| / 7\'7   Xilinx XC4000XV I/O Buffer IBIS File
| \ \   Xilinx Inc.
| / /   2100 Logic Drive
| \_\/.\   San Jose,   CA 95124
| IBIS file xc4kxv.ibs created by s2ibis2 version 1.1
| North Carolina State University Electronics Research Laboratory  1995
[IBIS ver]   2.1
[File name]   xc4kxv.ibs
[File Rev]   1.1
[Date]   Dec. 11, 1998
[Source]   Spice netlist
[Notes]   - Best/worse process data included in this ibis model
   - Control flag setting:
   SLW=0 - fast slew rate
   SLW=1 - slow slew rate
   PCI=0 - driving 3.3V PCI bus
   PCI=1 - driving 5.0V PCI bus
   5VT=0 - 5.0V tolerant input off
   5VT=1 - 5.0V tolerant input on
   - Created by Joey Jia x4437
[Disclaimer] The data in this model is derived from SPICE simulations
   using modeling information extracted from the target pro-
   cess. While a great deal of care has been take to provide
   information that is accurate, this model is considered
   preliminary as it has not been verified by actual silicon
   measurement. Treat the data in this model as preliminary
   until actual silicon verification is performed.
[Copyright]   Xilinx Inc. All right reserved
|   Component XC40110XV_BG325[SLW=0;PCI=0;5VT=0]
[Component]   XC40110XV_BG325[SLW=0;PCI=0;5VT=0]
[Manufacturer]   Xilinx Inc.
[Package]
| variable   typ   min   max
R_pkg   0.206   0.146   0.267
L_pkg   4.950nH   3.300nH   6.600nH
C_pkg   0.885pF   0.650pF   1.120pF
[Pin]  signal_name   model_name   R_pin   L_pin   C_pin
io   iob   IO_000   NA   NA   NA
|   Component XC40110XV_BG325[SLW=0;PCI=0;5VT=1]
[Component]   XC40110XV_BG325[SLW=0;PCI=0;5VT=1]
[Manufacturer]   Xilinx Inc.
[Package]
| variable   typ   min   max
R_pkg   0.206   0.146   0.267
L_pkg   4.950nH   3.300nH   6.600nH
C_pkg   0.885pF   0.650pF   1.120pF
[Pin]  signal_name   model_name   R_pin   L_pin   C_pin
io   iob   IO_001   NA   NA   NA
|   Component XC40110XV_BG325[SLW=0;PCI=1;5VT=0]
[Component]   XC40110XV_BG325[SLW=0;PCI=1;5VT=0]
[Manufacturer]   Xilinx Inc.
[Package]
| variable   typ   min   max
R_pkg   0.206   0.146   0.267
L_pkg   4.950nH   3.300nH   6.600nH
C_pkg   0.885pF   0.650pF   1.120pF
[Pin]  signal_name   model_name   R_pin   L_pin   C_pin
io   iob   IO_010   NA   NA   NA
|   Component XC40110XV_BG325[SLW=0;PCI=1;5VT=1]
[Component]   XC40110XV_BG325[SLW=0;PCI=1;5VT=1]
[Manufacturer]   Xilinx Inc.
[Package]
| variable   typ   min   max
R_pkg   0.206   0.146   0.267
L_pkg   4.950nH   3.300nH   6.600nH
C_pkg   0.885pF   0.650pF   1.120pF
[Pin]  signal_name   model_name   R_pin   L_pin   C_pin
io   iob   IO_011   NA   NA   NA
|   Component XC40110XV_BG325[SLW=1;PCI=0;5VT=0]
[Component]   XC40110XV_BG325[SLW=1;PCI=0;5VT=0]
[Manufacturer]   Xilinx Inc.
[Package]
| variable   typ   min   max
R_pkg   0.206   0.146   0.267
L_pkg   4.950nH   3.300nH   6.600nH
C_pkg   0.885pF   0.650pF   1.120pF
[Pin]  signal_name   model_name   R_pin   L_pin   C_pin
io   iob   IO_100   NA   NA   NA
|   Component XC40110XV_BG325[SLW=1;PCI=0;5VT=1]
[Component]   XC40110XV_BG325[SLW=1;PCI=0;5VT=1]
[Manufacturer]   Xilinx Inc.
[Package]
| variable   typ   min   max
R_pkg   0.206   0.146   0.267
L_pkg   4.950nH   3.300nH   6.600nH
C_pkg   0.885pF   0.650pF   1.120pF
[Pin]  signal_name   model_name   R_pin   L_pin   C_pin
io   iob   IO_101   NA   NA   NA
|   Component XC40110XV_BG325[SLW=1;PCI=1;5VT=0]
[Component]   XC40110XV_BG325[SLW=1;PCI=1;5VT=0]
[Manufacturer]   Xilinx Inc.
[Package]
| variable   typ   min   max
R_pkg   0.206   0.146   0.267
L_pkg   4.950nH   3.300nH   6.600nH
C_pkg   0.885pF   0.650pF   1.120pF
[Pin]  signal_name   model_name   R_pin   L_pin   C_pin
io   iob   IO_110   NA   NA   NA
|   Component XC40110XV_BG325[SLW=1;PCI=1;5VT=1]
[Component]   XC40110XV_BG325[SLW=1;PCI=1;5VT=1]
[Manufacturer]   Xilinx Inc.
[Package]
| variable   typ   min   max
R_pkg   0.206   0.146   0.267
L_pkg   4.950nH   3.300nH   6.600nH
C_pkg   0.885pF   0.650pF   1.120pF
[Pin]  signal_name   model_name   R_pin   L_pin   C_pin
io   iob   IO_111   NA   NA   NA
|+++++++++++++++++++++++++++++++++++++++++++++++++++++++++++++++++++++++++
|   Component XC40110XV_BG432[SLW=0;PCI=0;5VT=0]
[Component]   XC40110XV_BG432[SLW=0;PCI=0;5VT=0]
[Manufacturer]   Xilinx Inc.
[Package]
| variable   typ   min   max
R_pkg   249.500m   187.000m   312.000m
L_pkg   6.200nH   4.500nH   7.900nH
C_pkg   1.100pF   0.850pF   1.350pF
[Pin]  signal_name   model_name   R_pin   L_pin   C_pin
io   iob   IO_000   NA   NA   NA
| End [Component] XC40110XV_BG432[SLW=0;PCI=0;5VT=0]
|   Component XC40110XV_BG432[SLW=0;PCI=0;5VT=1]
[Component]   XC40110XV_BG432[SLW=0;PCI=0;5VT=1]
[Manufacturer]   Xilinx Inc.
[Package]
| variable   typ   min   max
R_pkg   249.500m   187.000m   312.000m
L_pkg   6.200nH   4.500nH   7.900nH
C_pkg   1.100pF   0.850pF   1.350pF
[Pin]  signal_name   model_name   R_pin   L_pin   C_pin
io   iob   IO_001   NA   NA   NA
| End [Component] XC40110XV_BG432[SLW=0;PCI=0;5VT=1]
|   Component XC40110XV_BG432[SLW=0;PCI=1;5VT=0]
[Component]   XC40110XV_BG432[SLW=0;PCI=1;5VT=0]
[Manufacturer]   Xilinx Inc.
[Package]
| variable   typ   min   max
R_pkg   249.500m   187.000m   312.000m
L_pkg   6.200nH   4.500nH   7.900nH
C_pkg   1.100pF   0.850pF   1.350pF
[Pin]  signal_name   model_name   R_pin   L_pin   C_pin
io   iob   IO_010   NA   NA   NA
| End [Component] XC40110XV_BG432[SLW=0;PCI=1;5VT=0]
|   Component XC40110XV_BG432[SLW=0;PCI=1;5VT=1]
[Component]   XC40110XV_BG432[SLW=0;PCI=1;5VT=1]
[Manufacturer]   Xilinx Inc.
[Package]
| variable   typ   min   max
R_pkg   249.500m   187.000m   312.000m
L_pkg   6.200nH   4.500nH   7.900nH
C_pkg   1.100pF   0.850pF   1.350pF
[Pin]  signal_name   model_name   R_pin   L_pin   C_pin
io   iob   IO_011   NA   NA   NA
| End [Component] XC40110XV_BG432[SLW=0;PCI=1;5VT=1]
|   Component XC40110XV_BG432[SLW=1;PCI=0;5VT=0]
[Component]   XC40110XV_BG432[SLW=1;PCI=0;5VT=0]
[Manufacturer]   Xilinx Inc.
[Package]
| variable   typ   min   max
R_pkg   249.500m   187.000m   312.000m
L_pkg   6.200nH   4.500nH   7.900nH
C_pkg   1.100pF   0.850pF   1.350pF
[Pin]  signal_name   model_name   R_pin   L_pin   C_pin
io   iob   IO_100   NA   NA   NA
| End [Component] XC40110XV_BG432[SLW=1;PCI=0;5VT=0]
|   Component XC40110XV_BG432[SLW=1;PCI=0;5VT=1]
[Component]   XC40110XV_BG432[SLW=1;PCI=0;5VT=1]
[Manufacturer]   Xilinx Inc.
[Package]
| variable   typ   min   max
R_pkg   249.500m   187.000m   312.000m
L_pkg   6.200nH   4.500nH   7.900nH
C_pkg   1.100pF   0.850pF   1.350pF
[Pin]  signal_name   model_name   R_pin   L_pin   C_pin
io   iob   IO_101   NA   NA   NA
| End [Component] XC40110XV_BG432[SLW=1;PCI=0;5VT=1]
|   Component XC40110XV_BG432[SLW=1;PCI=1;5VT=0]
[Component]   XC40110XV_BG432[SLW=1;PCI=1;5VT=0]
[Manufacturer]   Xilinx Inc.
[Package]
| variable   typ   min   max
R_pkg   249.500m   187.000m   312.000m
L_pkg   6.200nH   4.500nH   7.900nH
C_pkg   1.100pF   0.850pF   1.350pF
[Pin]  signal_name   model_name   R_pin   L_pin   C_pin
io   iob   IO_110   NA   NA   NA
| End [Component] XC40110XV_BG432[SLW=1;PCI=1;5VT=0]
|   Component XC40110XV_BG432[SLW=1;PCI=1;5VT=1]
[Component]   XC40110XV_BG432[SLW=1;PCI=1;5VT=1]
[Manufacturer]   Xilinx Inc.
[Package]
| variable   typ   min   max
R_pkg   249.500m   187.000m   312.000m
L_pkg   6.200nH   4.500nH   7.900nH
C_pkg   1.100pF   0.850pF   1.350pF
[Pin]  signal_name   model_name   R_pin   L_pin   C_pin
io   iob   IO_111   NA   NA   NA
| End [Component] XC40110XV_BG432[SLW=1;PCI=1;5VT=1]
|+++++++++++++++++++++++++++++++++++++++++++++++++++++++++++++++++++++++++
|   Component XC40110XV_BG560[SLW=0;PCI=0;5VT=0]
[Component]   XC40110XV_BG560[SLW=0;PCI=0;5VT=0]
[Manufacturer]   Xilinx Inc.
[Package]
| variable   typ   min   max
R_pkg   247.500m   172.000m   323.000m
L_pkg   6.150nH   4.100nH   8.200nH
C_pkg   1.090pF   0.780pF   1.400pF
[Pin]  signal_name   model_name   R_pin   L_pin   C_pin
io   iob   IO_000   NA   NA   NA
| End [Component] XC40110XV_BG560[SLW=0;PCI=0;5VT=0]
|   Component XC40110XV_BG560[SLW=0;PCI=0;5VT=1]
[Component]   XC40110XV_BG560[SLW=0;PCI=0;5VT=1]
[Manufacturer]   Xilinx Inc.
[Package]
| variable   typ   min   max
R_pkg   247.500m   172.000m   323.000m
L_pkg   6.150nH   4.100nH   8.200nH
C_pkg   1.090pF   0.780pF   1.400pF
[Pin]  signal_name   model_name   R_pin   L_pin   C_pin
io   iob   IO_001   NA   NA   NA
| End [Component] XC40110XV_BG560[SLW=0;PCI=0;5VT=1]
|   Component XC40110XV_BG560[SLW=0;PCI=1;5VT=0]
[Component]   XC40110XV_BG560[SLW=0;PCI=1;5VT=0]
[Manufacturer]   Xilinx Inc.
[Package]
| variable   typ   min   max
R_pkg   247.500m   172.000m   323.000m
L_pkg   6.150nH   4.100nH   8.200nH
C_pkg   1.090pF   0.780pF   1.400pF
[Pin]  signal_name   model_name   R_pin   L_pin   C_pin
io   iob   IO_010   NA   NA   NA
| End [Component] XC40110XV_BG560[SLW=0;PCI=1;5VT=0]
|   Component XC40110XV_BG560[SLW=0;PCI=1;5VT=1]
[Component]   XC40110XV_BG560[SLW=0;PCI=1;5VT=1]
[Manufacturer]   Xilinx Inc.
[Package]
| variable   typ   min   max
R_pkg   247.500m   172.000m   323.000m
L_pkg   6.150nH   4.100nH   8.200nH
C_pkg   1.090pF   0.780pF   1.400pF
[Pin]  signal_name   model_name   R_pin   L_pin   C_pin
io   iob   IO_011   NA   NA   NA
| End [Component] XC40110XV_BG560[SLW=0;PCI=1;5VT=1]
|   Component XC40110XV_BG560[SLW=1;PCI=0;5VT=0]
[Component]   XC40110XV_BG560[SLW=1;PCI=0;5VT=0]
[Manufacturer]   Xilinx Inc.
[Package]
| variable   typ   min   max
R_pkg   247.500m   172.000m   323.000m
L_pkg   6.150nH   4.100nH   8.200nH
C_pkg   1.090pF   0.780pF   1.400pF
[Pin]  signal_name   model_name   R_pin   L_pin   C_pin
io   iob   IO_100   NA   NA   NA
| End [Component] XC40110XV_BG560[SLW=1;PCI=0;5VT=0]
|   Component XC40110XV_BG560[SLW=1;PCI=0;5VT=1]
[Component]   XC40110XV_BG560[SLW=1;PCI=0;5VT=1]
[Manufacturer]   Xilinx Inc.
[Package]
| variable   typ   min   max
R_pkg   247.500m   172.000m   323.000m
L_pkg   6.150nH   4.100nH   8.200nH
C_pkg   1.090pF   0.780pF   1.400pF
[Pin]  signal_name   model_name   R_pin   L_pin   C_pin
io   iob   IO_101   NA   NA   NA
| End [Component] XC40110XV_BG560[SLW=1;PCI=0;5VT=1]
|   Component XC40110XV_BG560[SLW=1;PCI=1;5VT=0]
[Component]   XC40110XV_BG560[SLW=1;PCI=1;5VT=0]
[Manufacturer]   Xilinx Inc.
[Package]
| variable   typ   min   max
R_pkg   247.500m   172.000m   323.000m
L_pkg   6.150nH   4.100nH   8.200nH
C_pkg   1.090pF   0.780pF   1.400pF
[Pin]  signal_name   model_name   R_pin   L_pin   C_pin
io   iob   IO_110   NA   NA   NA
| End [Component] XC40110XV_BG560[SLW=1;PCI=1;5VT=0]
|   Component XC40110XV_BG560[SLW=1;PCI=1;5VT=1]
[Component]   XC40110XV_BG560[SLW=1;PCI=1;5VT=1]
[Manufacturer]   Xilinx Inc.
[Package]
| variable   typ   min   max
R_pkg   247.500m   172.000m   323.000m
L_pkg   6.150nH   4.100nH   8.200nH
C_pkg   1.090pF   0.780pF   1.400pF
[Pin]  signal_name   model_name   R_pin   L_pin   C_pin
io   iob   IO_111   NA   NA   NA
| End [Component] XC40110XV_BG560[SLW=1;PCI=1;5VT=1]
|+++++++++++++++++++++++++++++++++++++++++++++++++++++++++++++++++++++++++
|   Component XC40110XV_HQ240[SLW=0;PCI=0;5VT=0]
[Component]   XC40110XV_HQ240[SLW=0;PCI=0;5VT=0]
[Manufacturer]   Xilinx Inc.
[Package]
| variable   typ   min   max
R_pkg   185.500m   172.000m   198.000m
L_pkg   9.150nH   7.800nH   10.500nH
C_pkg   1.380pF   1.180pF   1.580pF
[Pin]  signal_name   model_name   R_pin   L_pin   C_pin
io   iob   IO_000   NA   NA   NA
| End [Component] XC40110XV_HQ240[SLW=0;PCI=0;5VT=0]
|   Component XC40110XV_HQ240[SLW=0;PCI=0;5VT=1]
[Component]   XC40110XV_HQ240[SLW=0;PCI=0;5VT=1]
[Manufacturer]   Xilinx Inc.
[Package]
| variable   typ   min   max
R_pkg   185.500m   172.000m   198.000m
L_pkg   9.150nH   7.800nH   10.500nH
C_pkg   1.380pF   1.180pF   1.580pF
[Pin]  signal_name   model_name   R_pin   L_pin   C_pin
io   iob   IO_001   NA   NA   NA
| End [Component] XC40110XV_HQ240[SLW=0;PCI=0;5VT=1]
|   Component XC40110XV_HQ240[SLW=0;PCI=1;5VT=0]
[Component]   XC40110XV_HQ240[SLW=0;PCI=1;5VT=0]
[Manufacturer]   Xilinx Inc.
[Package]
| variable   typ   min   max
R_pkg   185.500m   172.000m   198.000m
L_pkg   9.150nH   7.800nH   10.500nH
C_pkg   1.380pF   1.180pF   1.580pF
[Pin]  signal_name   model_name   R_pin   L_pin   C_pin
io   iob   IO_010   NA   NA   NA
| End [Component] XC40110XV_HQ240[SLW=0;PCI=1;5VT=0]
|   Component XC40110XV_HQ240[SLW=0;PCI=1;5VT=1]
[Component]   XC40110XV_HQ240[SLW=0;PCI=1;5VT=1]
[Manufacturer]   Xilinx Inc.
[Package]
| variable   typ   min   max
R_pkg   185.500m   172.000m   198.000m
L_pkg   9.150nH   7.800nH   10.500nH
C_pkg   1.380pF   1.180pF   1.580pF
[Pin]  signal_name   model_name   R_pin   L_pin   C_pin
io   iob   IO_011   NA   NA   NA
| End [Component] XC40110XV_HQ240[SLW=0;PCI=1;5VT=1]
|   Component XC40110XV_HQ240[SLW=1;PCI=0;5VT=0]
[Component]   XC40110XV_HQ240[SLW=1;PCI=0;5VT=0]
[Manufacturer]   Xilinx Inc.
[Package]
| variable   typ   min   max
R_pkg   185.500m   172.000m   198.000m
L_pkg   9.150nH   7.800nH   10.500nH
C_pkg   1.380pF   1.180pF   1.580pF
[Pin]  signal_name   model_name   R_pin   L_pin   C_pin
io   iob   IO_100   NA   NA   NA
| End [Component] XC40110XV_HQ240[SLW=1;PCI=0;5VT=0]
|   Component XC40110XV_HQ240[SLW=1;PCI=0;5VT=1]
[Component]   XC40110XV_HQ240[SLW=1;PCI=0;5VT=1]
[Manufacturer]   Xilinx Inc.
[Package]
| variable   typ   min   max
R_pkg   185.500m   172.000m   198.000m
L_pkg   9.150nH   7.800nH   10.500nH
C_pkg   1.380pF   1.180pF   1.580pF
[Pin]  signal_name   model_name   R_pin   L_pin   C_pin
io   iob   IO_101   NA   NA   NA
| End [Component] XC40110XV_HQ240[SLW=1;PCI=0;5VT=1]
|   Component XC40110XV_HQ240[SLW=1;PCI=1;5VT=0]
[Component]   XC40110XV_HQ240[SLW=1;PCI=1;5VT=0]
[Manufacturer]   Xilinx Inc.
[Package]
| variable   typ   min   max
R_pkg   185.500m   172.000m   198.000m
L_pkg   9.150nH   7.800nH   10.500nH
C_pkg   1.380pF   1.180pF   1.580pF
[Pin]  signal_name   model_name   R_pin   L_pin   C_pin
io   iob   IO_110   NA   NA   NA
| End [Component] XC40110XV_HQ240[SLW=1;PCI=1;5VT=0]
|   Component XC40110XV_HQ240[SLW=1;PCI=1;5VT=1]
[Component]   XC40110XV_HQ240[SLW=1;PCI=1;5VT=1]
[Manufacturer]   Xilinx Inc.
[Package]
| variable   typ   min   max
R_pkg   185.500m   172.000m   198.000m
L_pkg   9.150nH   7.800nH   10.500nH
C_pkg   1.380pF   1.180pF   1.580pF
[Pin]  signal_name   model_name   R_pin   L_pin   C_pin
io   iob   IO_111   NA   NA   NA
| End [Component] XC40110XV_HQ240[SLW=1;PCI=1;5VT=1]
|+++++++++++++++++++++++++++++++++++++++++++++++++++++++++++++++++++++++++
|   Component XC40150XV_BG432[SLW=0;PCI=0;5VT=0]
[Component]   XC40150XV_BG432[SLW=0;PCI=0;5VT=0]
[Manufacturer]   Xilinx Inc.
[Package]
| variable   typ   min   max
R_pkg   240.500m   180.000m   301.000m
L_pkg   5.950nH   4.300nH   7.600nH
C_pkg   1.050pF   0.810pF   1.290pF
[Pin]  signal_name   model_name   R_pin   L_pin   C_pin
io   iob   IO_000   NA   NA   NA
| End [Component] XC40150XV_BG432[SLW=0;PCI=0;5VT=0]
|   Component XC40150XV_BG432[SLW=0;PCI=0;5VT=1]
[Component]   XC40150XV_BG432[SLW=0;PCI=0;5VT=1]
[Manufacturer]   Xilinx Inc.
[Package]
| variable   typ   min   max
R_pkg   240.500m   180.000m   301.000m
L_pkg   5.950nH   4.300nH   7.600nH
C_pkg   1.050pF   0.810pF   1.290pF
[Pin]  signal_name   model_name   R_pin   L_pin   C_pin
io   iob   IO_001   NA   NA   NA
| End [Component] XC40150XV_BG432[SLW=0;PCI=0;5VT=1]
|   Component XC40150XV_BG432[SLW=0;PCI=1;5VT=0]
[Component]   XC40150XV_BG432[SLW=0;PCI=1;5VT=0]
[Manufacturer]   Xilinx Inc.
[Package]
| variable   typ   min   max
R_pkg   240.500m   180.000m   301.000m
L_pkg   5.950nH   4.300nH   7.600nH
C_pkg   1.050pF   0.810pF   1.290pF
[Pin]  signal_name   model_name   R_pin   L_pin   C_pin
io   iob   IO_010   NA   NA   NA
| End [Component] XC40150XV_BG432[SLW=0;PCI=1;5VT=0]
|   Component XC40150XV_BG432[SLW=0;PCI=1;5VT=1]
[Component]   XC40150XV_BG432[SLW=0;PCI=1;5VT=1]
[Manufacturer]   Xilinx Inc.
[Package]
| variable   typ   min   max
R_pkg   240.500m   180.000m   301.000m
L_pkg   5.950nH   4.300nH   7.600nH
C_pkg   1.050pF   0.810pF   1.290pF
[Pin]  signal_name   model_name   R_pin   L_pin   C_pin
io   iob   IO_011   NA   NA   NA
| End [Component] XC40150XV_BG432[SLW=0;PCI=1;5VT=1]
|   Component XC40150XV_BG432[SLW=1;PCI=0;5VT=0]
[Component]   XC40150XV_BG432[SLW=1;PCI=0;5VT=0]
[Manufacturer]   Xilinx Inc.
[Package]
| variable   typ   min   max
R_pkg   240.500m   180.000m   301.000m
L_pkg   5.950nH   4.300nH   7.600nH
C_pkg   1.050pF   0.810pF   1.290pF
[Pin]  signal_name   model_name   R_pin   L_pin   C_pin
io   iob   IO_100   NA   NA   NA
| End [Component] XC40150XV_BG432[SLW=1;PCI=0;5VT=0]
|   Component XC40150XV_BG432[SLW=1;PCI=0;5VT=1]
[Component]   XC40150XV_BG432[SLW=1;PCI=0;5VT=1]
[Manufacturer]   Xilinx Inc.
[Package]
| variable   typ   min   max
R_pkg   240.500m   180.000m   301.000m
L_pkg   5.950nH   4.300nH   7.600nH
C_pkg   1.050pF   0.810pF   1.290pF
[Pin]  signal_name   model_name   R_pin   L_pin   C_pin
io   iob   IO_101   NA   NA   NA
| End [Component] XC40150XV_BG432[SLW=1;PCI=0;5VT=1]
|   Component XC40150XV_BG432[SLW=1;PCI=1;5VT=0]
[Component]   XC40150XV_BG432[SLW=1;PCI=1;5VT=0]
[Manufacturer]   Xilinx Inc.
[Package]
| variable   typ   min   max
R_pkg   240.500m   180.000m   301.000m
L_pkg   5.950nH   4.300nH   7.600nH
C_pkg   1.050pF   0.810pF   1.290pF
[Pin]  signal_name   model_name   R_pin   L_pin   C_pin
io   iob   IO_110   NA   NA   NA
| End [Component] XC40150XV_BG432[SLW=1;PCI=1;5VT=0]
|   Component XC40150XV_BG432[SLW=1;PCI=1;5VT=1]
[Component]   XC40150XV_BG432[SLW=1;PCI=1;5VT=1]
[Manufacturer]   Xilinx Inc.
[Package]
| variable   typ   min   max
R_pkg   240.500m   180.000m   301.000m
L_pkg   5.950nH   4.300nH   7.600nH
C_pkg   1.050pF   0.810pF   1.290pF
[Pin]  signal_name   model_name   R_pin   L_pin   C_pin
io   iob   IO_111   NA   NA   NA
| End [Component] XC40150XV_BG432[SLW=1;PCI=1;5VT=1]
|+++++++++++++++++++++++++++++++++++++++++++++++++++++++++++++++++++++++++
|   Component XC40150XV_BG560[SLW=0;PCI=0;5VT=0]
[Component]   XC40150XV_BG560[SLW=0;PCI=0;5VT=0]
[Manufacturer]   Xilinx Inc.
[Package]
| variable   typ   min   max
R_pkg   249.000m   180.000m   318.000m
L_pkg   6.150nH   4.300nH   8.000nH
C_pkg   1.095pF   0.810pF   1.380pF
[Pin]  signal_name   model_name   R_pin   L_pin   C_pin
io   iob   IO_000   NA   NA   NA
| End [Component] XC40150XV_BG560[SLW=0;PCI=0;5VT=0]
|   Component XC40150XV_BG560[SLW=0;PCI=0;5VT=1]
[Component]   XC40150XV_BG560[SLW=0;PCI=0;5VT=1]
[Manufacturer]   Xilinx Inc.
[Package]
| variable   typ   min   max
R_pkg   249.000m   180.000m   318.000m
L_pkg   6.150nH   4.300nH   8.000nH
C_pkg   1.095pF   0.810pF   1.380pF
[Pin]  signal_name   model_name   R_pin   L_pin   C_pin
io   iob   IO_001   NA   NA   NA
| End [Component] XC40150XV_BG560[SLW=0;PCI=0;5VT=1]
|   Component XC40150XV_BG560[SLW=0;PCI=1;5VT=0]
[Component]   XC40150XV_BG560[SLW=0;PCI=1;5VT=0]
[Manufacturer]   Xilinx Inc.
[Package]
| variable   typ   min   max
R_pkg   249.000m   180.000m   318.000m
L_pkg   6.150nH   4.300nH   8.000nH
C_pkg   1.095pF   0.810pF   1.380pF
[Pin]  signal_name   model_name   R_pin   L_pin   C_pin
io   iob   IO_010   NA   NA   NA
| End [Component] XC40150XV_BG560[SLW=0;PCI=1;5VT=0]
|   Component XC40150XV_BG560[SLW=0;PCI=1;5VT=1]
[Component]   XC40150XV_BG560[SLW=0;PCI=1;5VT=1]
[Manufacturer]   Xilinx Inc.
[Package]
| variable   typ   min   max
R_pkg   249.000m   180.000m   318.000m
L_pkg   6.150nH   4.300nH   8.000nH
C_pkg   1.095pF   0.810pF   1.380pF
[Pin]  signal_name   model_name   R_pin   L_pin   C_pin
io   iob   IO_011   NA   NA   NA
| End [Component] XC40150XV_BG560[SLW=0;PCI=1;5VT=1]
|   Component XC40150XV_BG560[SLW=1;PCI=0;5VT=0]
[Component]   XC40150XV_BG560[SLW=1;PCI=0;5VT=0]
[Manufacturer]   Xilinx Inc.
[Package]
| variable   typ   min   max
R_pkg   249.000m   180.000m   318.000m
L_pkg   6.150nH   4.300nH   8.000nH
C_pkg   1.095pF   0.810pF   1.380pF
[Pin]  signal_name   model_name   R_pin   L_pin   C_pin
io   iob   IO_100   NA   NA   NA
| End [Component] XC40150XV_BG560[SLW=1;PCI=0;5VT=0]
|   Component XC40150XV_BG560[SLW=1;PCI=0;5VT=1]
[Component]   XC40150XV_BG560[SLW=1;PCI=0;5VT=1]
[Manufacturer]   Xilinx Inc.
[Package]
| variable   typ   min   max
R_pkg   249.000m   180.000m   318.000m
L_pkg   6.150nH   4.300nH   8.000nH
C_pkg   1.095pF   0.810pF   1.380pF
[Pin]  signal_name   model_name   R_pin   L_pin   C_pin
io   iob   IO_101   NA   NA   NA
| End [Component] XC40150XV_BG560[SLW=1;PCI=0;5VT=1]
|   Component XC40150XV_BG560[SLW=1;PCI=1;5VT=0]
[Component]   XC40150XV_BG560[SLW=1;PCI=1;5VT=0]
[Manufacturer]   Xilinx Inc.
[Package]
| variable   typ   min   max
R_pkg   249.000m   180.000m   318.000m
L_pkg   6.150nH   4.300nH   8.000nH
C_pkg   1.095pF   0.810pF   1.380pF
[Pin]  signal_name   model_name   R_pin   L_pin   C_pin
io   iob   IO_110   NA   NA   NA
| End [Component] XC40150XV_BG560[SLW=1;PCI=1;5VT=0]
|   Component XC40150XV_BG560[SLW=1;PCI=1;5VT=1]
[Component]   XC40150XV_BG560[SLW=1;PCI=1;5VT=1]
[Manufacturer]   Xilinx Inc.
[Package]
| variable   typ   min   max
R_pkg   249.000m   180.000m   318.000m
L_pkg   6.150nH   4.300nH   8.000nH
C_pkg   1.095pF   0.810pF   1.380pF
[Pin]  signal_name   model_name   R_pin   L_pin   C_pin
io   iob   IO_111   NA   NA   NA
| End [Component] XC40150XV_BG560[SLW=1;PCI=1;5VT=1]
|+++++++++++++++++++++++++++++++++++++++++++++++++++++++++++++++++++++++++
|   Component XC40150XV_HQ240[SLW=0;PCI=0;5VT=0]
[Component]   XC40150XV_HQ240[SLW=0;PCI=0;5VT=0]
[Manufacturer]   Xilinx Inc.
[Package]
| variable   typ   min   max
R_pkg   160.500m   149.000m   172.000m
L_pkg   7.950nH   6.800nH   9.100nH
C_pkg   1.200pF   1.000pF   1.400pF
[Pin]  signal_name   model_name   R_pin   L_pin   C_pin
io   iob   IO_000   NA   NA   NA
| End [Component] XC40150XV_HQ240[SLW=0;PCI=0;5VT=0]
|   Component XC40150XV_HQ240[SLW=0;PCI=0;5VT=1]
[Component]   XC40150XV_HQ240[SLW=0;PCI=0;5VT=1]
[Manufacturer]   Xilinx Inc.
[Package]
| variable   typ   min   max
R_pkg   160.500m   149.000m   172.000m
L_pkg   7.950nH   6.800nH   9.100nH
C_pkg   1.200pF   1.000pF   1.400pF
[Pin]  signal_name   model_name   R_pin   L_pin   C_pin
io   iob   IO_001   NA   NA   NA
| End [Component] XC40150XV_HQ240[SLW=0;PCI=0;5VT=1]
|   Component XC40150XV_HQ240[SLW=0;PCI=1;5VT=0]
[Component]   XC40150XV_HQ240[SLW=0;PCI=1;5VT=0]
[Manufacturer]   Xilinx Inc.
[Package]
| variable   typ   min   max
R_pkg   160.500m   149.000m   172.000m
L_pkg   7.950nH   6.800nH   9.100nH
C_pkg   1.200pF   1.000pF   1.400pF
[Pin]  signal_name   model_name   R_pin   L_pin   C_pin
io   iob   IO_010   NA   NA   NA
| End [Component] XC40150XV_HQ240[SLW=0;PCI=1;5VT=0]
|   Component XC40150XV_HQ240[SLW=0;PCI=1;5VT=1]
[Component]   XC40150XV_HQ240[SLW=0;PCI=1;5VT=1]
[Manufacturer]   Xilinx Inc.
[Package]
| variable   typ   min   max
R_pkg   160.500m   149.000m   172.000m
L_pkg   7.950nH   6.800nH   9.100nH
C_pkg   1.200pF   1.000pF   1.400pF
[Pin]  signal_name   model_name   R_pin   L_pin   C_pin
io   iob   IO_011   NA   NA   NA
| End [Component] XC40150XV_HQ240[SLW=0;PCI=1;5VT=1]
|   Component XC40150XV_HQ240[SLW=1;PCI=0;5VT=0]
[Component]   XC40150XV_HQ240[SLW=1;PCI=0;5VT=0]
[Manufacturer]   Xilinx Inc.
[Package]
| variable   typ   min   max
R_pkg   160.500m   149.000m   172.000m
L_pkg   7.950nH   6.800nH   9.100nH
C_pkg   1.200pF   1.000pF   1.400pF
[Pin]  signal_name   model_name   R_pin   L_pin   C_pin
io   iob   IO_100   NA   NA   NA
| End [Component] XC40150XV_HQ240[SLW=1;PCI=0;5VT=0]
|   Component XC40150XV_HQ240[SLW=1;PCI=0;5VT=1]
[Component]   XC40150XV_HQ240[SLW=1;PCI=0;5VT=1]
[Manufacturer]   Xilinx Inc.
[Package]
| variable   typ   min   max
R_pkg   160.500m   149.000m   172.000m
L_pkg   7.950nH   6.800nH   9.100nH
C_pkg   1.200pF   1.000pF   1.400pF
[Pin]  signal_name   model_name   R_pin   L_pin   C_pin
io   iob   IO_101   NA   NA   NA
| End [Component] XC40150XV_HQ240[SLW=1;PCI=0;5VT=1]
|   Component XC40150XV_HQ240[SLW=1;PCI=1;5VT=0]
[Component]   XC40150XV_HQ240[SLW=1;PCI=1;5VT=0]
[Manufacturer]   Xilinx Inc.
[Package]
| variable   typ   min   max
R_pkg   160.500m   149.000m   172.000m
L_pkg   7.950nH   6.800nH   9.100nH
C_pkg   1.200pF   1.000pF   1.400pF
[Pin]  signal_name   model_name   R_pin   L_pin   C_pin
io   iob   IO_110   NA   NA   NA
| End [Component] XC40150XV_HQ240[SLW=1;PCI=1;5VT=0]
|   Component XC40150XV_HQ240[SLW=1;PCI=1;5VT=1]
[Component]   XC40150XV_HQ240[SLW=1;PCI=1;5VT=1]
[Manufacturer]   Xilinx Inc.
[Package]
| variable   typ   min   max
R_pkg   160.500m   149.000m   172.000m
L_pkg   7.950nH   6.800nH   9.100nH
C_pkg   1.200pF   1.000pF   1.400pF
[Pin]  signal_name   model_name   R_pin   L_pin   C_pin
io   iob   IO_111   NA   NA   NA
| End [Component] XC40150XV_HQ240[SLW=1;PCI=1;5VT=1]
|+++++++++++++++++++++++++++++++++++++++++++++++++++++++++++++++++++++++++
|   Component XC40200XV_BG432[SLW=0;PCI=0;5VT=0]
[Component]   XC40200XV_BG432[SLW=0;PCI=0;5VT=0]
[Manufacturer]   Xilinx Inc.
[Package]
| variable   typ   min   max
R_pkg   221.500m   164.000m   279.000m
L_pkg   5.350nH   3.800nH   6.900nH
C_pkg   0.960pF   0.740pF   1.180pF
[Pin]  signal_name   model_name   R_pin   L_pin   C_pin
io   iob   IO_000   NA   NA   NA
| End [Component] XC40200XV_BG432[SLW=0;PCI=0;5VT=0]
|   Component XC40200XV_BG432[SLW=0;PCI=0;5VT=1]
[Component]   XC40200XV_BG432[SLW=0;PCI=0;5VT=1]
[Manufacturer]   Xilinx Inc.
[Package]
| variable   typ   min   max
R_pkg   221.500m   164.000m   279.000m
L_pkg   5.350nH   3.800nH   6.900nH
C_pkg   0.960pF   0.740pF   1.180pF
[Pin]  signal_name   model_name   R_pin   L_pin   C_pin
io   iob   IO_001   NA   NA   NA
| End [Component] XC40200XV_BG432[SLW=0;PCI=0;5VT=1]
|   Component XC40200XV_BG432[SLW=0;PCI=1;5VT=0]
[Component]   XC40200XV_BG432[SLW=0;PCI=1;5VT=0]
[Manufacturer]   Xilinx Inc.
[Package]
| variable   typ   min   max
R_pkg   221.500m   164.000m   279.000m
L_pkg   5.350nH   3.800nH   6.900nH
C_pkg   0.960pF   0.740pF   1.180pF
[Pin]  signal_name   model_name   R_pin   L_pin   C_pin
io   iob   IO_010   NA   NA   NA
| End [Component] XC40200XV_BG432[SLW=0;PCI=1;5VT=0]
|   Component XC40200XV_BG432[SLW=0;PCI=1;5VT=1]
[Component]   XC40200XV_BG432[SLW=0;PCI=1;5VT=1]
[Manufacturer]   Xilinx Inc.
[Package]
| variable   typ   min   max
R_pkg   221.500m   164.000m   279.000m
L_pkg   5.350nH   3.800nH   6.900nH
C_pkg   0.960pF   0.740pF   1.180pF
[Pin]  signal_name   model_name   R_pin   L_pin   C_pin
io   iob   IO_011   NA   NA   NA
| End [Component] XC40200XV_BG432[SLW=0;PCI=1;5VT=1]
|   Component XC40200XV_BG432[SLW=1;PCI=0;5VT=0]
[Component]   XC40200XV_BG432[SLW=1;PCI=0;5VT=0]
[Manufacturer]   Xilinx Inc.
[Package]
| variable   typ   min   max
R_pkg   221.500m   164.000m   279.000m
L_pkg   5.350nH   3.800nH   6.900nH
C_pkg   0.960pF   0.740pF   1.180pF
[Pin]  signal_name   model_name   R_pin   L_pin   C_pin
io   iob   IO_100   NA   NA   NA
| End [Component] XC40200XV_BG432[SLW=1;PCI=0;5VT=0]
|   Component XC40200XV_BG432[SLW=1;PCI=0;5VT=1]
[Component]   XC40200XV_BG432[SLW=1;PCI=0;5VT=1]
[Manufacturer]   Xilinx Inc.
[Package]
| variable   typ   min   max
R_pkg   221.500m   164.000m   279.000m
L_pkg   5.350nH   3.800nH   6.900nH
C_pkg   0.960pF   0.740pF   1.180pF
[Pin]  signal_name   model_name   R_pin   L_pin   C_pin
io   iob   IO_101   NA   NA   NA
| End [Component] XC40200XV_BG432[SLW=1;PCI=0;5VT=1]
|   Component XC40200XV_BG432[SLW=1;PCI=1;5VT=0]
[Component]   XC40200XV_BG432[SLW=1;PCI=1;5VT=0]
[Manufacturer]   Xilinx Inc.
[Package]
| variable   typ   min   max
R_pkg   221.500m   164.000m   279.000m
L_pkg   5.350nH   3.800nH   6.900nH
C_pkg   0.960pF   0.740pF   1.180pF
[Pin]  signal_name   model_name   R_pin   L_pin   C_pin
io   iob   IO_110   NA   NA   NA
| End [Component] XC40200XV_BG432[SLW=1;PCI=1;5VT=0]
|   Component XC40200XV_BG432[SLW=1;PCI=1;5VT=1]
[Component]   XC40200XV_BG432[SLW=1;PCI=1;5VT=1]
[Manufacturer]   Xilinx Inc.
[Package]
| variable   typ   min   max
R_pkg   221.500m   164.000m   279.000m
L_pkg   5.350nH   3.800nH   6.900nH
C_pkg   0.960pF   0.740pF   1.180pF
[Pin]  signal_name   model_name   R_pin   L_pin   C_pin
io   iob   IO_111   NA   NA   NA
| End [Component] XC40200XV_BG432[SLW=1;PCI=1;5VT=1]
|+++++++++++++++++++++++++++++++++++++++++++++++++++++++++++++++++++++++++
|   Component XC40200XV_BG560[SLW=0;PCI=0;5VT=0]
[Component]   XC40200XV_BG560[SLW=0;PCI=0;5VT=0]
[Manufacturer]   Xilinx Inc.
[Package]
| variable   typ   min   max
R_pkg   232.000m   164.000m   300.000m
L_pkg   5.700nH   3.900nH   7.500nH
C_pkg   1.015pF   0.740pF   1.290pF
[Pin]  signal_name   model_name   R_pin   L_pin   C_pin
io   iob   IO_000   NA   NA   NA
| End [Component] XC40200XV_BG560[SLW=0;PCI=0;5VT=0]
|   Component XC40200XV_BG560[SLW=0;PCI=0;5VT=1]
[Component]   XC40200XV_BG560[SLW=0;PCI=0;5VT=1]
[Manufacturer]   Xilinx Inc.
[Package]
| variable   typ   min   max
R_pkg   232.000m   164.000m   300.000m
L_pkg   5.700nH   3.900nH   7.500nH
C_pkg   1.015pF   0.740pF   1.290pF
[Pin]  signal_name   model_name   R_pin   L_pin   C_pin
io   iob   IO_001   NA   NA   NA
| End [Component] XC40200XV_BG560[SLW=0;PCI=0;5VT=1]
|   Component XC40200XV_BG560[SLW=0;PCI=1;5VT=0]
[Component]   XC40200XV_BG560[SLW=0;PCI=1;5VT=0]
[Manufacturer]   Xilinx Inc.
[Package]
| variable   typ   min   max
R_pkg   232.000m   164.000m   300.000m
L_pkg   5.700nH   3.900nH   7.500nH
C_pkg   1.015pF   0.740pF   1.290pF
[Pin]  signal_name   model_name   R_pin   L_pin   C_pin
io   iob   IO_010   NA   NA   NA
| End [Component] XC40200XV_BG560[SLW=0;PCI=1;5VT=0]
|   Component XC40200XV_BG560[SLW=0;PCI=1;5VT=1]
[Component]   XC40200XV_BG560[SLW=0;PCI=1;5VT=1]
[Manufacturer]   Xilinx Inc.
[Package]
| variable   typ   min   max
R_pkg   232.000m   164.000m   300.000m
L_pkg   5.700nH   3.900nH   7.500nH
C_pkg   1.015pF   0.740pF   1.290pF
[Pin]  signal_name   model_name   R_pin   L_pin   C_pin
io   iob   IO_011   NA   NA   NA
| End [Component] XC40200XV_BG560[SLW=0;PCI=1;5VT=1]
|   Component XC40200XV_BG560[SLW=1;PCI=0;5VT=0]
[Component]   XC40200XV_BG560[SLW=1;PCI=0;5VT=0]
[Manufacturer]   Xilinx Inc.
[Package]
| variable   typ   min   max
R_pkg   232.000m   164.000m   300.000m
L_pkg   5.700nH   3.900nH   7.500nH
C_pkg   1.015pF   0.740pF   1.290pF
[Pin]  signal_name   model_name   R_pin   L_pin   C_pin
io   iob   IO_100   NA   NA   NA
| End [Component] XC40200XV_BG560[SLW=1;PCI=0;5VT=0]
|   Component XC40200XV_BG560[SLW=1;PCI=0;5VT=1]
[Component]   XC40200XV_BG560[SLW=1;PCI=0;5VT=1]
[Manufacturer]   Xilinx Inc.
[Package]
| variable   typ   min   max
R_pkg   232.000m   164.000m   300.000m
L_pkg   5.700nH   3.900nH   7.500nH
C_pkg   1.015pF   0.740pF   1.290pF
[Pin]  signal_name   model_name   R_pin   L_pin   C_pin
io   iob   IO_101   NA   NA   NA
| End [Component] XC40200XV_BG560[SLW=1;PCI=0;5VT=1]
|   Component XC40200XV_BG560[SLW=1;PCI=1;5VT=0]
[Component]   XC40200XV_BG560[SLW=1;PCI=1;5VT=0]
[Manufacturer]   Xilinx Inc.
[Package]
| variable   typ   min   max
R_pkg   232.000m   164.000m   300.000m
L_pkg   5.700nH   3.900nH   7.500nH
C_pkg   1.015pF   0.740pF   1.290pF
[Pin]  signal_name   model_name   R_pin   L_pin   C_pin
io   iob   IO_110   NA   NA   NA
| End [Component] XC40200XV_BG560[SLW=1;PCI=1;5VT=0]
|   Component XC40200XV_BG560[SLW=1;PCI=1;5VT=1]
[Component]   XC40200XV_BG560[SLW=1;PCI=1;5VT=1]
[Manufacturer]   Xilinx Inc.
[Package]
| variable   typ   min   max
R_pkg   232.000m   164.000m   300.000m
L_pkg   5.700nH   3.900nH   7.500nH
C_pkg   1.015pF   0.740pF   1.290pF
[Pin]  signal_name   model_name   R_pin   L_pin   C_pin
io   iob   IO_111   NA   NA   NA
| End [Component] XC40200XV_BG560[SLW=1;PCI=1;5VT=1]
|+++++++++++++++++++++++++++++++++++++++++++++++++++++++++++++++++++++++++
|   Component XC40200XV_HQ240[SLW=0;PCI=0;5VT=0]
[Component]   XC40200XV_HQ240[SLW=0;PCI=0;5VT=0]
[Manufacturer]   Xilinx Inc.
[Package]
| variable   typ   min   max
R_pkg   160.500m   149.000m   172.000m
L_pkg   7.950nH   6.800nH   9.100nH
C_pkg   1.200pF   1.000pF   1.400pF
[Pin]  signal_name   model_name   R_pin   L_pin   C_pin
io   iob   IO_000   NA   NA   NA
| End [Component] XC40200XV_HQ240[SLW=0;PCI=0;5VT=0]
|   Component XC40200XV_HQ240[SLW=0;PCI=0;5VT=1]
[Component]   XC40200XV_HQ240[SLW=0;PCI=0;5VT=1]
[Manufacturer]   Xilinx Inc.
[Package]
| variable   typ   min   max
R_pkg   160.500m   149.000m   172.000m
L_pkg   7.950nH   6.800nH   9.100nH
C_pkg   1.200pF   1.000pF   1.400pF
[Pin]  signal_name   model_name   R_pin   L_pin   C_pin
io   iob   IO_001   NA   NA   NA
| End [Component] XC40200XV_HQ240[SLW=0;PCI=0;5VT=1]
|   Component XC40200XV_HQ240[SLW=0;PCI=1;5VT=0]
[Component]   XC40200XV_HQ240[SLW=0;PCI=1;5VT=0]
[Manufacturer]   Xilinx Inc.
[Package]
| variable   typ   min   max
R_pkg   160.500m   149.000m   172.000m
L_pkg   7.950nH   6.800nH   9.100nH
C_pkg   1.200pF   1.000pF   1.400pF
[Pin]  signal_name   model_name   R_pin   L_pin   C_pin
io   iob   IO_010   NA   NA   NA
| End [Component] XC40200XV_HQ240[SLW=0;PCI=1;5VT=0]
|   Component XC40200XV_HQ240[SLW=0;PCI=1;5VT=1]
[Component]   XC40200XV_HQ240[SLW=0;PCI=1;5VT=1]
[Manufacturer]   Xilinx Inc.
[Package]
| variable   typ   min   max
R_pkg   160.500m   149.000m   172.000m
L_pkg   7.950nH   6.800nH   9.100nH
C_pkg   1.200pF   1.000pF   1.400pF
[Pin]  signal_name   model_name   R_pin   L_pin   C_pin
io   iob   IO_011   NA   NA   NA
| End [Component] XC40200XV_HQ240[SLW=0;PCI=1;5VT=1]
|   Component XC40200XV_HQ240[SLW=1;PCI=0;5VT=0]
[Component]   XC40200XV_HQ240[SLW=1;PCI=0;5VT=0]
[Manufacturer]   Xilinx Inc.
[Package]
| variable   typ   min   max
R_pkg   160.500m   149.000m   172.000m
L_pkg   7.950nH   6.800nH   9.100nH
C_pkg   1.200pF   1.000pF   1.400pF
[Pin]  signal_name   model_name   R_pin   L_pin   C_pin
io   iob   IO_100   NA   NA   NA
| End [Component] XC40200XV_HQ240[SLW=1;PCI=0;5VT=0]
|   Component XC40200XV_HQ240[SLW=1;PCI=0;5VT=1]
[Component]   XC40200XV_HQ240[SLW=1;PCI=0;5VT=1]
[Manufacturer]   Xilinx Inc.
[Package]
| variable   typ   min   max
R_pkg   160.500m   149.000m   172.000m
L_pkg   7.950nH   6.800nH   9.100nH
C_pkg   1.200pF   1.000pF   1.400pF
[Pin]  signal_name   model_name   R_pin   L_pin   C_pin
io   iob   IO_101   NA   NA   NA
| End [Component] XC40200XV_HQ240[SLW=1;PCI=0;5VT=1]
|   Component XC40200XV_HQ240[SLW=1;PCI=1;5VT=0]
[Component]   XC40200XV_HQ240[SLW=1;PCI=1;5VT=0]
[Manufacturer]   Xilinx Inc.
[Package]
| variable   typ   min   max
R_pkg   160.500m   149.000m   172.000m
L_pkg   7.950nH   6.800nH   9.100nH
C_pkg   1.200pF   1.000pF   1.400pF
[Pin]  signal_name   model_name   R_pin   L_pin   C_pin
io   iob   IO_110   NA   NA   NA
| End [Component] XC40200XV_HQ240[SLW=1;PCI=1;5VT=0]
|   Component XC40200XV_HQ240[SLW=1;PCI=1;5VT=1]
[Component]   XC40200XV_HQ240[SLW=1;PCI=1;5VT=1]
[Manufacturer]   Xilinx Inc.
[Package]
| variable   typ   min   max
R_pkg   160.500m   149.000m   172.000m
L_pkg   7.950nH   6.800nH   9.100nH
C_pkg   1.200pF   1.000pF   1.400pF
[Pin]  signal_name   model_name   R_pin   L_pin   C_pin
io   iob   IO_111   NA   NA   NA
| End [Component] XC40200XV_HQ240[SLW=1;PCI=1;5VT=1]
|+++++++++++++++++++++++++++++++++++++++++++++++++++++++++++++++++++++++++
|   Component XC40250XV_BG432[SLW=0;PCI=0;5VT=0]
[Component]   XC40250XV_BG432[SLW=0;PCI=0;5VT=0]
[Manufacturer]   Xilinx Inc.
[Package]
| variable   typ   min   max
R_pkg   221.500m   164.000m   279.000m
L_pkg   5.350nH   3.800nH   6.900nH
C_pkg   0.960pF   0.740pF   1.180pF
[Pin]  signal_name   model_name   R_pin   L_pin   C_pin
io   iob   IO_000   NA   NA   NA
| End [Component] XC40250XV_BG432[SLW=0;PCI=0;5VT=0]
|   Component XC40250XV_BG432[SLW=0;PCI=0;5VT=1]
[Component]   XC40250XV_BG432[SLW=0;PCI=0;5VT=1]
[Manufacturer]   Xilinx Inc.
[Package]
| variable   typ   min   max
R_pkg   221.500m   164.000m   279.000m
L_pkg   5.350nH   3.800nH   6.900nH
C_pkg   0.960pF   0.740pF   1.180pF
[Pin]  signal_name   model_name   R_pin   L_pin   C_pin
io   iob   IO_001   NA   NA   NA
| End [Component] XC40250XV_BG432[SLW=0;PCI=0;5VT=1]
|   Component XC40250XV_BG432[SLW=0;PCI=1;5VT=0]
[Component]   XC40250XV_BG432[SLW=0;PCI=1;5VT=0]
[Manufacturer]   Xilinx Inc.
[Package]
| variable   typ   min   max
R_pkg   221.500m   164.000m   279.000m
L_pkg   5.350nH   3.800nH   6.900nH
C_pkg   0.960pF   0.740pF   1.180pF
[Pin]  signal_name   model_name   R_pin   L_pin   C_pin
io   iob   IO_010   NA   NA   NA
| End [Component] XC40250XV_BG432[SLW=0;PCI=1;5VT=0]
|   Component XC40250XV_BG432[SLW=0;PCI=1;5VT=1]
[Component]   XC40250XV_BG432[SLW=0;PCI=1;5VT=1]
[Manufacturer]   Xilinx Inc.
[Package]
| variable   typ   min   max
R_pkg   221.500m   164.000m   279.000m
L_pkg   5.350nH   3.800nH   6.900nH
C_pkg   0.960pF   0.740pF   1.180pF
[Pin]  signal_name   model_name   R_pin   L_pin   C_pin
io   iob   IO_011   NA   NA   NA
| End [Component] XC40250XV_BG432[SLW=0;PCI=1;5VT=1]
|   Component XC40250XV_BG432[SLW=1;PCI=0;5VT=0]
[Component]   XC40250XV_BG432[SLW=1;PCI=0;5VT=0]
[Manufacturer]   Xilinx Inc.
[Package]
| variable   typ   min   max
R_pkg   221.500m   164.000m   279.000m
L_pkg   5.350nH   3.800nH   6.900nH
C_pkg   0.960pF   0.740pF   1.180pF
[Pin]  signal_name   model_name   R_pin   L_pin   C_pin
io   iob   IO_100   NA   NA   NA
| End [Component] XC40250XV_BG432[SLW=1;PCI=0;5VT=0]
|   Component XC40250XV_BG432[SLW=1;PCI=0;5VT=1]
[Component]   XC40250XV_BG432[SLW=1;PCI=0;5VT=1]
[Manufacturer]   Xilinx Inc.
[Package]
| variable   typ   min   max
R_pkg   221.500m   164.000m   279.000m
L_pkg   5.350nH   3.800nH   6.900nH
C_pkg   0.960pF   0.740pF   1.180pF
[Pin]  signal_name   model_name   R_pin   L_pin   C_pin
io   iob   IO_101   NA   NA   NA
| End [Component] XC40250XV_BG432[SLW=1;PCI=0;5VT=1]
|   Component XC40250XV_BG432[SLW=1;PCI=1;5VT=0]
[Component]   XC40250XV_BG432[SLW=1;PCI=1;5VT=0]
[Manufacturer]   Xilinx Inc.
[Package]
| variable   typ   min   max
R_pkg   221.500m   164.000m   279.000m
L_pkg   5.350nH   3.800nH   6.900nH
C_pkg   0.960pF   0.740pF   1.180pF
[Pin]  signal_name   model_name   R_pin   L_pin   C_pin
io   iob   IO_110   NA   NA   NA
| End [Component] XC40250XV_BG432[SLW=1;PCI=1;5VT=0]
|   Component XC40250XV_BG432[SLW=1;PCI=1;5VT=1]
[Component]   XC40250XV_BG432[SLW=1;PCI=1;5VT=1]
[Manufacturer]   Xilinx Inc.
[Package]
| variable   typ   min   max
R_pkg   221.500m   164.000m   279.000m
L_pkg   5.350nH   3.800nH   6.900nH
C_pkg   0.960pF   0.740pF   1.180pF
[Pin]  signal_name   model_name   R_pin   L_pin   C_pin
io   iob   IO_111   NA   NA   NA
| End [Component] XC40250XV_BG432[SLW=1;PCI=1;5VT=1]
|+++++++++++++++++++++++++++++++++++++++++++++++++++++++++++++++++++++++++
|   Component XC40250XV_BG560[SLW=0;PCI=0;5VT=0]
[Component]   XC40250XV_BG560[SLW=0;PCI=0;5VT=0]
[Manufacturer]   Xilinx Inc.
[Package]
| variable   typ   min   max
R_pkg   232.000m   164.000m   300.000m
L_pkg   5.700nH   3.900nH   7.500nH
C_pkg   1.015pF   0.740pF   1.290pF
[Pin]  signal_name   model_name   R_pin   L_pin   C_pin
io   iob   IO_000   NA   NA   NA
| End [Component] XC40250XV_BG560[SLW=0;PCI=0;5VT=0]
|   Component XC40250XV_BG560[SLW=0;PCI=0;5VT=1]
[Component]   XC40250XV_BG560[SLW=0;PCI=0;5VT=1]
[Manufacturer]   Xilinx Inc.
[Package]
| variable   typ   min   max
R_pkg   232.000m   164.000m   300.000m
L_pkg   5.700nH   3.900nH   7.500nH
C_pkg   1.015pF   0.740pF   1.290pF
[Pin]  signal_name   model_name   R_pin   L_pin   C_pin
io   iob   IO_001   NA   NA   NA
| End [Component] XC40250XV_BG560[SLW=0;PCI=0;5VT=1]
|   Component XC40250XV_BG560[SLW=0;PCI=1;5VT=0]
[Component]   XC40250XV_BG560[SLW=0;PCI=1;5VT=0]
[Manufacturer]   Xilinx Inc.
[Package]
| variable   typ   min   max
R_pkg   232.000m   164.000m   300.000m
L_pkg   5.700nH   3.900nH   7.500nH
C_pkg   1.015pF   0.740pF   1.290pF
[Pin]  signal_name   model_name   R_pin   L_pin   C_pin
io   iob   IO_010   NA   NA   NA
| End [Component] XC40250XV_BG560[SLW=0;PCI=1;5VT=0]
|   Component XC40250XV_BG560[SLW=0;PCI=1;5VT=1]
[Component]   XC40250XV_BG560[SLW=0;PCI=1;5VT=1]
[Manufacturer]   Xilinx Inc.
[Package]
| variable   typ   min   max
R_pkg   232.000m   164.000m   300.000m
L_pkg   5.700nH   3.900nH   7.500nH
C_pkg   1.015pF   0.740pF   1.290pF
[Pin]  signal_name   model_name   R_pin   L_pin   C_pin
io   iob   IO_011   NA   NA   NA
| End [Component] XC40250XV_BG560[SLW=0;PCI=1;5VT=1]
|   Component XC40250XV_BG560[SLW=1;PCI=0;5VT=0]
[Component]   XC40250XV_BG560[SLW=1;PCI=0;5VT=0]
[Manufacturer]   Xilinx Inc.
[Package]
| variable   typ   min   max
R_pkg   232.000m   164.000m   300.000m
L_pkg   5.700nH   3.900nH   7.500nH
C_pkg   1.015pF   0.740pF   1.290pF
[Pin]  signal_name   model_name   R_pin   L_pin   C_pin
io   iob   IO_100   NA   NA   NA
| End [Component] XC40250XV_BG560[SLW=1;PCI=0;5VT=0]
|   Component XC40250XV_BG560[SLW=1;PCI=0;5VT=1]
[Component]   XC40250XV_BG560[SLW=1;PCI=0;5VT=1]
[Manufacturer]   Xilinx Inc.
[Package]
| variable   typ   min   max
R_pkg   232.000m   164.000m   300.000m
L_pkg   5.700nH   3.900nH   7.500nH
C_pkg   1.015pF   0.740pF   1.290pF
[Pin]  signal_name   model_name   R_pin   L_pin   C_pin
io   iob   IO_101   NA   NA   NA
| End [Component] XC40250XV_BG560[SLW=1;PCI=0;5VT=1]
|   Component XC40250XV_BG560[SLW=1;PCI=1;5VT=0]
[Component]   XC40250XV_BG560[SLW=1;PCI=1;5VT=0]
[Manufacturer]   Xilinx Inc.
[Package]
| variable   typ   min   max
R_pkg   232.000m   164.000m   300.000m
L_pkg   5.700nH   3.900nH   7.500nH
C_pkg   1.015pF   0.740pF   1.290pF
[Pin]  signal_name   model_name   R_pin   L_pin   C_pin
io   iob   IO_110   NA   NA   NA
| End [Component] XC40250XV_BG560[SLW=1;PCI=1;5VT=0]
|   Component XC40250XV_BG560[SLW=1;PCI=1;5VT=1]
[Component]   XC40250XV_BG560[SLW=1;PCI=1;5VT=1]
[Manufacturer]   Xilinx Inc.
[Package]
| variable   typ   min   max
R_pkg   232.000m   164.000m   300.000m
L_pkg   5.700nH   3.900nH   7.500nH
C_pkg   1.015pF   0.740pF   1.290pF
[Pin]  signal_name   model_name   R_pin   L_pin   C_pin
io   iob   IO_111   NA   NA   NA
| End [Component] XC40250XV_BG560[SLW=1;PCI=1;5VT=1]
| Models and submodels in the file (8): IO_000 (I/O), IO_001 (I/O), IO_010 (I/O), IO_011 (I/O), IO_100 (I/O), IO_101 (I/O), IO_110 (I/O), IO_111 (I/O)
